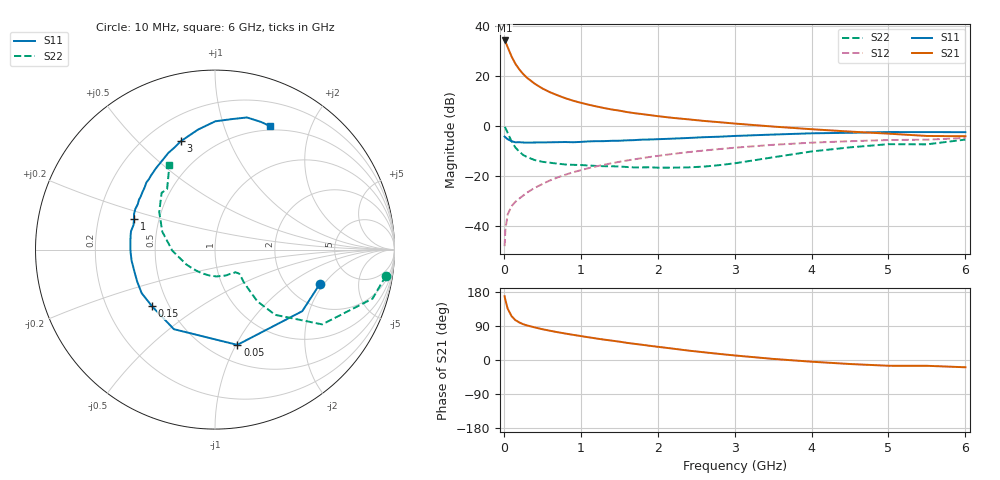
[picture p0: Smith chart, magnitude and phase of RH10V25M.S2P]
! SIEMENS Small Signal Semiconductors
! BFR106
! Si NPN RF Bipolar Junction Transistor in SOT23
! VCE = 10 V  IC = 25 mA
! Common Emitter S-Parameters:  August  1996
# GHz  S  MA  R  50
!  f  S11  S21  S12  S22
! GHz  MAG  ANG  MAG  ANG  MAG  ANG  MAG  ANG
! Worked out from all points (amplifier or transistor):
!   36 points, 10 MHz to 6 GHz, reference 50 ohm
!   highest |S21| = 34.1 dB at 10 MHz (marker M1)
!   |S21| within 3 dB of that: start of sweep to 54.15 MHz
!   unconditionally stable (mu >= 1): 362.9 MHz to 2.14 GHz
!   at 250 MHz: K = 0.91, MSG = 24.3 dB, |S12| = -27.8 dB
!   at 1.4 GHz: K = 1.06, MAG = 9.2 dB, |S12| = -14.9 dB
!   at 6 GHz: K = 0.98, MSG = 0.3 dB, |S12| = -4.8 dB
!   S11 on the Smith chart (normalised r, x): 10 MHz: 2.97, -1.82; 50 MHz: 0.67, -1.01; 150 MHz: 0.40, -0.33; 1 GHz: 0.36, +0.16; 3 GHz: 0.34, +0.68; 6 GHz: 0.45, +1.44
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0.01  0.6147 -18.1  50.96 168.1  0.004 83.6  0.9635 -8.7
0.02  0.5951 -35.2  48.23 158.6  0.0085 76.9  0.9191 -17.3
0.05  0.5452 -76.8  37.36 135.5  0.0172 61.8  0.7282 -34.9
0.1  0.4991 -117.3  24.51 115.8  0.0252 55.9  0.4947 -47.3
0.15  0.4722 -138.0  17.45 105.2  0.0307 55.5  0.3727 -50.7
0.2  0.4752 -149.4  13.55 99.2  0.0356 58.5  0.3089 -50.0
0.25  0.4687 -157.6  10.95 94.5  0.0407 60.9  0.2649 -49.2
0.3  0.4656 -163.7  9.215 91.3  0.0467 62.7  0.2407 -48.5
0.4  0.4687 -172.4  7.004 86.1  0.0582 65.2  0.2096 -46.2
0.5  0.4708 -178.5  5.624 81.3  0.0694 66.9  0.1931 -44.9
0.6  0.4728 175.9  4.721 77.2  0.0821 67.6  0.1849 -45.5
0.8  0.479 167.8  3.584 69.8  0.1067 67.4  0.1708 -47.8
1  0.4818 159.5  2.908 63.2  0.1311 66.6  0.1664 -51.9
1.1  0.4929 156.2  2.667 60.0  0.1438 65.8  0.1631 -55.0
1.3  0.499 149.7  2.289 53.9  0.1684 64.0  0.1578 -61.0
1.6  0.5172 141.0  1.9 45.3  0.205 60.9  0.1521 -72.9
2.2  0.5602 125.9  1.451 29.9  0.2775 53.7  0.1475 -102.9
3  0.6332 107.5  1.12 12.0  0.369 42.6  0.1801 -152.8
3.5  0.675 98.1  0.975 2.9  0.4215 35.3  0.2375 -178.4
4.5  0.7323 82.9  0.774 -10.6  0.4975 20.0  0.3752 145.9
5.5  0.756 70.1  0.633 -15.3  0.5342 9.2  0.4305 128.3
6  0.7531 65.9  0.625 -19.2  0.5768 1.7  0.5366 118.2
